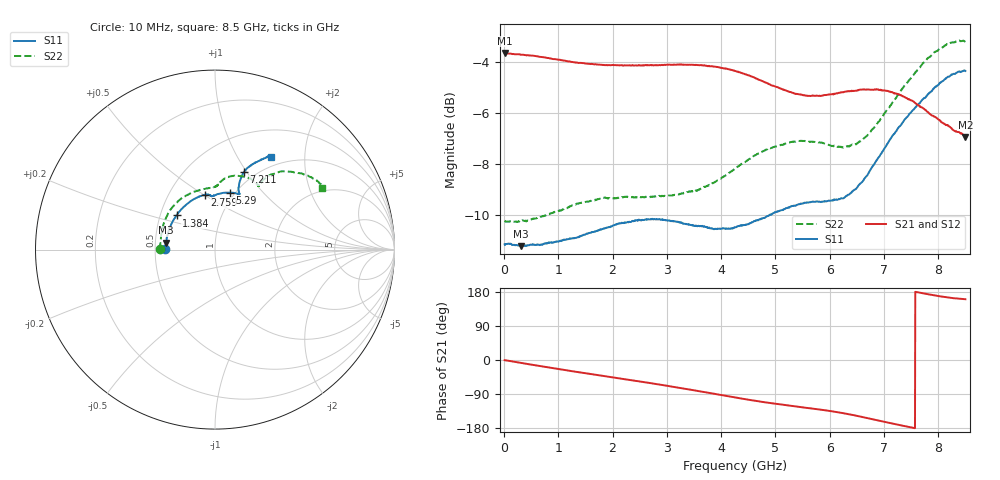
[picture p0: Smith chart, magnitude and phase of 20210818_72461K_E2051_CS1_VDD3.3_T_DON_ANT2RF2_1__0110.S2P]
!Agilent Technologies,E5071C,MY46417908,A.11.23
!Date: Wed Aug 18 14:26:53 2021
!Data & Calibration Information:
!Freq	S11:SOLT2(ON)	S21:SOLT2(ON)	S12:SOLT2(ON)	S22:SOLT2(ON)
!PortZ  Port1:50+j0  Port2:50+j0
!Above PortZ is port z conversion or system Z0 setting when saving the data.
!When reading, reference impedance value at option line is always used.
# Hz S dB R 50
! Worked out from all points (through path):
!   1601 points, 10 MHz to 8.5 GHz, reference 50 ohm
!   highest |S21| = -3.65 dB at 10 MHz (marker M1); lowest = -6.9 dB at 8.5 GHz (marker M2)
!   group delay of S21, straight-line fit = 65.1 ps
!   lowest |S11| = -11.2 dB at 312.5 MHz (marker M3), VSWR 1.76, Z = 28.5 + j2.41 ohm
!   |S11| at or under -10 dB: start of sweep to 4.886 GHz
!   |S22| runs from -10.3 to -3.2 dB; largest |S21 - S12| = 0.0023
!   S11 on the Smith chart (normalised r, x): 10 MHz: 0.57, +0.00; 1.384 GHz: 0.61, +0.25; 2.759 GHz: 0.75, +0.50; 5.29 GHz: 0.95, +0.68; 7.211 GHz: 0.89, +0.97; 8.5 GHz: 0.86, +1.40
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1e7  -11.15 179.6  -3.65 -0.4  -3.64 -0.4  -10.23 179.8
3.124562e8  -11.22 171.8  -3.72 -7.7  -3.71 -7.7  -10.24 171.3
9.385938e8  -11.06 153.8  -3.89 -22.5  -3.88 -22.5  -9.87 152.8
1.384319e9  -10.85 138.4  -4.04 -32.4  -4.04 -32.4  -9.54 138.0
1.426769e9  -10.81 136.9  -4.04 -33.3  -4.04 -33.3  -9.52 136.6
2.1325e9  -10.33 113.8  -4.13 -48.4  -4.13 -48.5  -9.33 113.4
2.758638e9  -10.17 100.5  -4.14 -62.4  -4.13 -62.4  -9.28 97.8
2.843538e9  -10.17 99.5  -4.12 -64.4  -4.12 -64.4  -9.26 96.5
3.591719e9  -10.43 94.3  -4.13 -82.3  -4.12 -82.3  -9.00 88.5
3.920706e9  -10.56 93.7  -4.20 -90.3  -4.20 -90.3  -8.66 86.5
4.255e9  -10.48 91.8  -4.35 -98.8  -4.35 -98.8  -8.19 83.7
4.748481e9  -10.15 86.1  -4.75 -110.4  -4.74 -110.4  -7.53 77.0
5.289719e9  -9.66 75.2  -5.19 -121.2  -5.20 -121.2  -7.14 66.9
5.671769e9  -9.49 68.7  -5.33 -128.0  -5.34 -128.0  -7.13 60.5
6.340356e9  -9.21 67.2  -5.14 -142.9  -5.15 -143.0  -7.30 55.4
6.796694e9  -8.07 69.9  -5.09 -156.4  -5.09 -156.5  -6.62 55.5
7.088538e9  -7.12 69.9  -5.15 -165.6  -5.16 -165.7  -5.80 53.8
7.210581e9  -6.75 69.5  -5.23 -169.3  -5.23 -169.3  -5.44 52.2
7.497119e9  -5.98 67.4  -5.51 -177.8  -5.51 -177.8  -4.64 48.0
7.985294e9  -4.92 62.4  -6.23 169.2  -6.20 169.3  -3.57 37.9
8.224075e9  -4.54 60.6  -6.56 164.1  -6.54 164.2  -3.26 33.5
8.5e9  -4.35 58.7  -6.94 160.4  -6.90 160.3  -3.21 30.0
